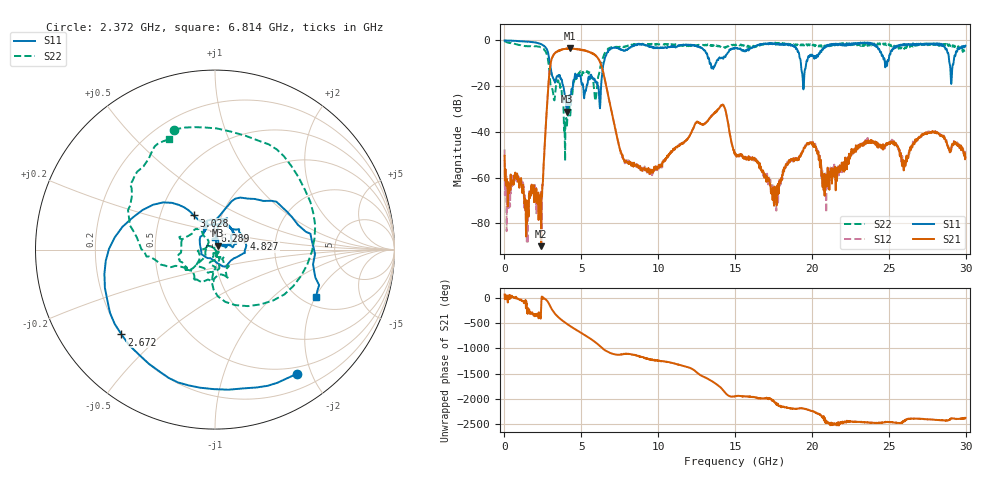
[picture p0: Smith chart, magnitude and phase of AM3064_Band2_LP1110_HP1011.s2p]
# Hz S DB R 50.0
!freq dBS11 angS11 dBS21 angS21 dBS12 angS12 dBS22 angS22
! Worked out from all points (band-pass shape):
!   1600 points, 10 MHz to 29.98 GHz, reference 50 ohm
!   highest |S21| = -3.46 dB at 4.246 GHz (marker M1); lowest = -90.0 dB at 2.39 GHz (marker M2)
!   |S21| within 3 dB of the highest: 3.187 GHz to 5.896 GHz (2.709 GHz wide, 59.6 % of centre)
!   lowest |S11| = -31.3 dB at 4.059 GHz (marker M3), VSWR 1.06, Z = 51.7 + j2.22 ohm
!   |S11| at or under -10 dB: 2.955 GHz to 6.45 GHz (3.496 GHz wide, 74.3 % of centre); 13.4 GHz to 13.74 GHz (338.3 MHz wide, 2.49 % of centre); 19.28 GHz to 19.62 GHz (342.2 MHz wide, 1.76 % of centre)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
!   |S22| runs from -52.7 to -0.3 dB; largest |S21 - S12| = 0.022
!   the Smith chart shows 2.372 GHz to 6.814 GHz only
!   S11 on the Smith chart (normalised r, x): 2.372 GHz: 0.40, -1.78; 2.672 GHz: 0.20, -0.37; 3.028 GHz: 0.74, +0.30; 4.827 GHz: 1.37, +0.17; 6.289 GHz: 0.97, +0.21; 6.814 GHz: 2.34, -2.03
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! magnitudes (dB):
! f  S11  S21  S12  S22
! 10 MHz  -0.1  -50.5  -47.7  -0.3
! 1.435 GHz  -0.5  -76.8  -79.8  -2.5
! 2.372 GHz  -1.6  -74.6  -66.2  -3.0
! 2.39 GHz  -1.7  -90.0  -67.6  -3.1
! 2.672 GHz  -3.1  -39.5  -39.5  -4.8
! 3.028 GHz  -13.0  -9.2  -9.2  -20.1
! 4.059 GHz  -31.3  -3.6  -3.5  -37.6
! 4.246 GHz  -24.1  -3.5  -3.6  -32.1
! 4.827 GHz  -15.3  -3.9  -3.9  -14.4
! 5.015 GHz  -18.7  -4.2  -4.1  -15.0
! 5.914 GHz  -18.4  -6.6  -6.6  -26.4
! 6.289 GHz  -19.5  -10.8  -10.7  -10.1
! 6.814 GHz  -4.1  -26.3  -26.3  -3.5
! 7.845 GHz  -4.5  -52.6  -52.6  -2.8
! 10 GHz  -3.4  -55.5  -54.7  -1.8
! 14.14 GHz  -7.6  -28.3  -28.4  -3.0
! 15 GHz  -3.3  -50.0  -49.7  -1.9
! 17.65 GHz  -1.9  -68.3  -67.2  -1.2
! 19.99 GHz  -6.3  -44.8  -44.9  -1.7
! 20.89 GHz  -2.5  -64.1  -65.2  -2.9
! 25 GHz  -8.4  -44.8  -45.1  -1.7
! 29.98 GHz  -2.4  -51.2  -51.9  -4.5
